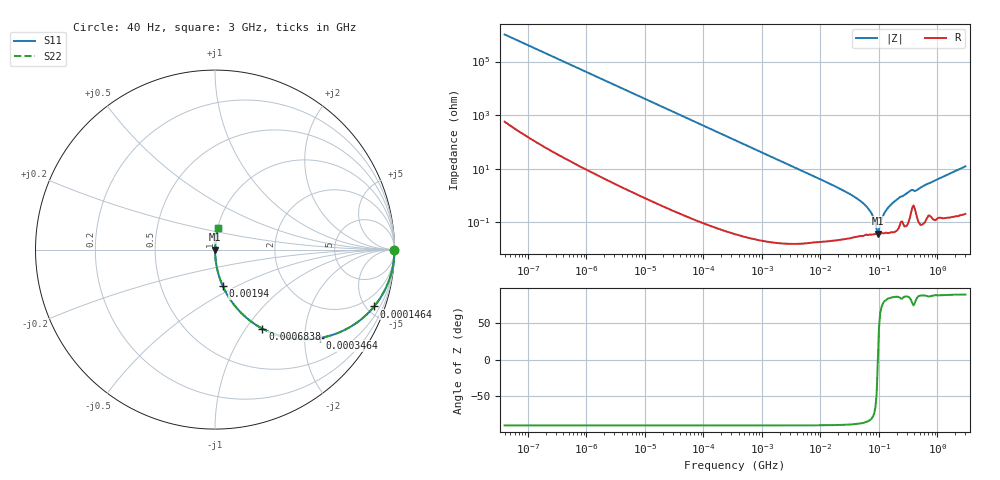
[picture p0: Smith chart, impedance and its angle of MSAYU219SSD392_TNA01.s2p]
! MSAYU219SSD392_TNA01  S-PARAMETER MODEL  ( General Type )
! Model Generated by TAIYO YUDEN Corporation (http://www.ty-top.com)
! Version 2.0
! TAIYO YUDEN Control No. 031016
! Copyright(c) 2003 TAIYO YUDEN CO.,LTD. All Rights Reserved.
! Product Description (link to TY-COMPAS)
! https://ds.yuden.co.jp/TYCOMPAS/or/detail?pn=MSAYU219SSD392KTNA01&u=M
! Products Name : Multilayer Ceramic Capacitors
! Characteristics :
!  Capacitance : 3900 pF , Rated Voltage : 50V
!  Case Size : 2.0 x 1.25 / 0.079 x 0.049 [mm/inch] , Thickness : 0.85 / 0.033 [mm/inch]
!  (Conditions: Temperature = 25 degC , DC Bias Current/Voltage = 0A / 0V)
! External Node Assignments :
!  1  o---| |---o  2
! GND o---------o GND
! Frequency Range : 40Hz  -  3GHz  [ 401 STEP ]
# MHz S RI R 50
! Freq[MHz].  S11 Real  S11 Imag  S21 Real  S21 Imag  S12 Real  S12 Imag  S22 Real  S22 Imag
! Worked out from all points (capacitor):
!   401 points, 40 Hz to 3 GHz, reference 50 ohm
!   read as one part in series: C = 3.88 nF near 44 Hz
!   lowest |Z| = 38.6 mohm at 95.69 MHz (marker M1)
!   series resonance near 95.8 MHz, so ESL is about 710 pH
!   S11 on the Smith chart (normalised r, x): 40 Hz: open; 146.4 kHz: 1.00, -5.60; 346.4 kHz: 1.00, -2.37; 683.8 kHz: 1.00, -1.20; 1.94 MHz: 1.00, -0.42; 3 GHz: 1.00, +0.25
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4e-05  1 -9.76e-05  6.4e-08 9.76e-05  6.4e-08 9.76e-05  1 -9.76e-05
0.000834  1 -0.00204  4.61e-06 0.00204  4.61e-06 0.00204  1 -0.00204
0.017386  0.9982 -0.0424  0.00181 0.0424  0.00181 0.0424  0.9982 -0.0424
0.056505  0.9813 -0.1353  0.0187 0.1353  0.0187 0.1353  0.9813 -0.1353
0.146395  0.8867 -0.3168  0.1133 0.3168  0.1133 0.3168  0.8867 -0.3168
0.34641  0.5831 -0.4929  0.4169 0.4929  0.4169 0.4929  0.5831 -0.4929
0.362475  0.5609 -0.4961  0.4391 0.4961  0.4391 0.4961  0.5609 -0.4961
0.683763  0.2643 -0.4407  0.7357 0.4407  0.7357 0.4407  0.2643 -0.4407
1.939641  0.0428 -0.2021  0.9572 0.2021  0.9572 0.2021  0.0428 -0.2021
7.222098  0.00335 -0.0562  0.9967 0.0562  0.9967 0.0562  0.00335 -0.0562
25.69909  0.000455 -0.0147  0.9995 0.0147  0.9995 0.0147  0.000455 -0.0147
48.47801  0.000352 -0.00624  0.9996 0.00624  0.9996 0.00624  0.000352 -0.00624
69.67004  0.000358 -0.00274  0.9996 0.00274  0.9996 0.00274  0.000358 -0.00274
79.8195  0.00036 -0.00154  0.9996 0.00154  0.9996 0.00154  0.00036 -0.00154
87.39454  0.000376 -0.000771  0.9996 0.000771  0.9996 0.000771  0.000376 -0.000771
95.68847  0.000385 -1.02e-05  0.9996 1.02e-05  0.9996 1.02e-05  0.000385 -1.02e-05
104.7695  0.000385 0.000757  0.9996 -0.000757  0.9996 -0.000757  0.000385 0.000757
125.5988  0.000402 0.00232  0.9996 -0.00232  0.9996 -0.00232  0.000402 0.00232
150.5692  0.000422 0.00397  0.9996 -0.00397  0.9996 -0.00397  0.000422 0.00397
340.4975  0.00183 0.0149  0.9982 -0.0149  0.9982 -0.0149  0.00183 0.0149
446.9303  0.00181 0.0161  0.9982 -0.0161  0.9982 -0.0161  0.00181 0.0161
3000  0.0169 0.1206  0.9831 -0.1206  0.9831 -0.1206  0.0169 0.1206
